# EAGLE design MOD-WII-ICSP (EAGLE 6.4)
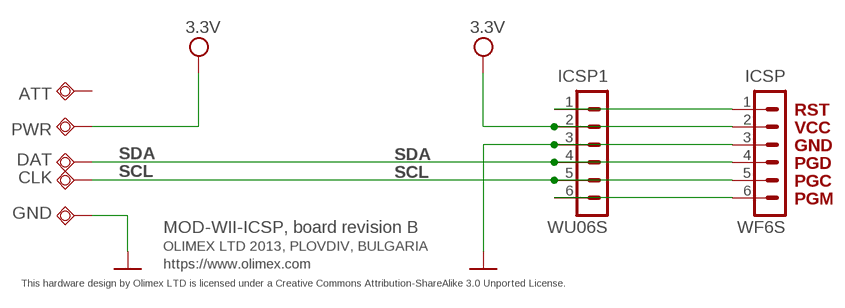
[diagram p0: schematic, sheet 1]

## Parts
ATT  TESTPADTESTPAD1.50X7.5MM  [TESTPAD1.50X7.5MM]
CLK  TESTPADTESTPAD1.50X7.5MM  [TESTPAD1.50X7.5MM]
DAT  TESTPADTESTPAD1.50X7.5MM  [TESTPAD1.50X7.5MM]
GND  TESTPADTESTPAD1.50X7.5MM  [TESTPAD1.50X7.5MM]
ICSP  WF6S  CON6WF6S  [WF6S]
ICSP1  WU06S  CON6WUO6S  [WU06S]
PWR  TESTPADTESTPAD1.50X7.5MM  [TESTPAD1.50X7.5MM]

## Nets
GND [pwr]: GND.1(PP) ICSP1.3 ICSP.3
N$1: ICSP1.1 ICSP.1
N$6: ICSP1.6 ICSP.6
SCL: CLK.1(PP) ICSP1.5 ICSP.5
SDA: DAT.1(PP) ICSP1.4 ICSP.4
VCC: ICSP1.2 ICSP.2 PWR.1(PP) ; supply symbol labelled 3.3V
Unconnected: ATT.1(PP)

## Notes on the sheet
- RST
- VCC
- GND
- PGD
- PGC
- PGM
- MOD-WII-ICSP, board revision B
- OLIMEX LTD 2013, PLOVDIV, BULGARIA
- https://www.olimex.com
- This hardware design by Olimex LTD is licensed under a Creative Commons Attribution-ShareAlike 3.0 Unported License.

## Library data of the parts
ATT CLK DAT GND PWR = gogo:TESTPAD: drill 40mils, diameter 70mils
ICSP ICSP1 = Penko:CON6: CONNECTORS - 6 PINS

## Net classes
1 pwr: width 0.25 mm

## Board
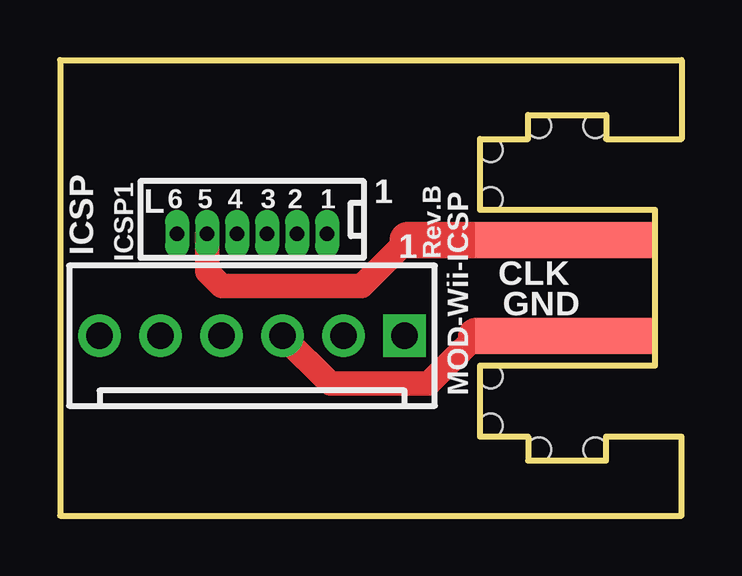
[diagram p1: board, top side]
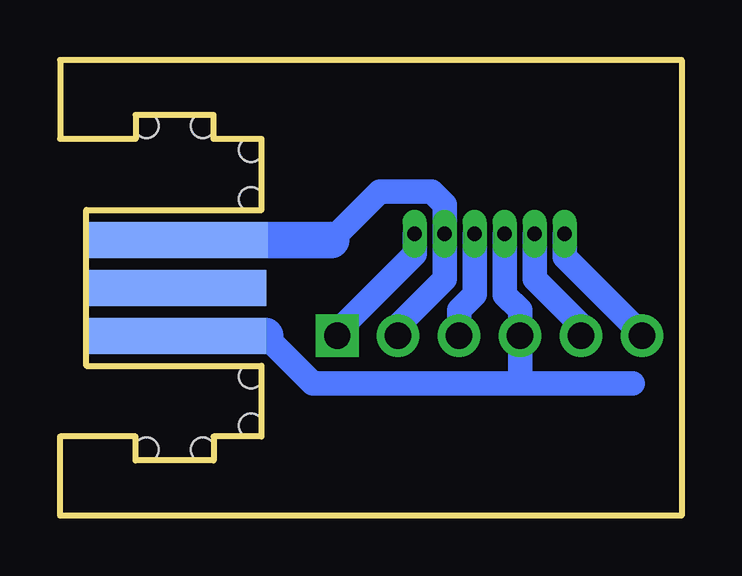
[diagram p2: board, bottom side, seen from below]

Size 25.9 x 19 mm. Coordinates in mm from the lower left corner, seen from the top.
Outline: 17.5,3.3 17.5,6.25 24.8,6.25 24.8,12.75 17.5,12.75 17.5,15.7 19.5,15.7 19.5,16.7 22.75,16.7 22.75,15.7 25.9,15.7 25.9,19 0,19 0,0 25.9,0 25.9,3.3 22.75,3.3 22.75,2.3 19.5,2.3 19.5,3.3 17.5,3.3
Copper layers (1+16): Top 0.035mm / dielectric 1.5mm / Bottom 0.035mm
Design rules "default": minimum track width 0.2mm, minimum drill 0.4mm, track to track 0.25mm, track to pad 0.25mm, pad to pad 0.25mm, via to via 0.25mm, smd to smd 1mil, copper to edge 10mil, drill to drill 8mil, minimum pad ring 8mil, minimum via ring 0.2mm, stop-mask expansion 4mil, vias tented up to drill 25mil, thermal gap 20mil
Holes 1 mm at 19.95,16.25 22.3,16.25 17.95,15.25 17.95,13.2 17.95,5.8 17.95,3.75 19.95,2.75 22.3,2.75

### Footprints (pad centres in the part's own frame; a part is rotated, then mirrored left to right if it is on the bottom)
TESTPAD1.50X7.5MM = smd 7.5 x 1.5: 1 0,0
WF6S = drill 1.1 pad 1.778 square: 1 -6.35,0 | drill 1.1 pad 1.778: 2 -3.81,0; 3 -1.27,0; 4 1.27,0; 5 3.81,0; 6 6.35,0
WU06S = drill 0.6 pad 0.991 long: 1 -3.125,0; 2 -1.875,0; 3 -0.625,0; 4 0.625,0; 5 1.875,0; 6 3.125,0

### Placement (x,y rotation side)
ATT  21.05,9.5 180 bottom
CLK  21.05,11.5 180 top
DAT  21.05,7.5 0 bottom
GND  21.05,7.5 0 top
ICSP  8,7.5 180 top
ICSP1  8,11.75 180 top
PWR  21,11.5 180 bottom

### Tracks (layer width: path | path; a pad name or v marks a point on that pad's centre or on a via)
GND
  Top 1.016: 17.35,7.5 15.37,5.52 11.25,5.52 ICSP.3
  Top 1.524: 17.35,7.5 GND.1
  Bottom 1.016: ICSP1.3 8.62,9.21 9.27,8.56 ICSP.3
N$1
  Bottom 1.016: ICSP1.1 11.12,10.9 14.35,7.68 ICSP.1
N$6
  Bottom 1.016: ICSP1.6 4.88,10.77 1.65,7.55 ICSP.6
SCL
  Top 1.016: 14.49,11.5 12.57,9.58 6.73,9.58 6.12,10.19 ICSP1.5
  Top 1.524: 14.49,11.5 CLK.1
  Bottom 1.016: ICSP1.5 6.12,9.86 4.19,7.93 ICSP.5
SDA
  Bottom 1.016: ICSP1.4 7.38,9.21 6.73,8.56 ICSP.4 6.73,7.29 6.73,5.52 | 17.35,7.5 15.37,5.52 6.73,5.52 | 6.73,5.52 6.1,5.52 | 2.03,5.52 6.73,5.52
  Bottom 1.524: 17.35,7.5 DAT.1
VCC
  Bottom 1.016: ICSP.2 11.81,7.93 9.88,9.87 ICSP1.2 9.88,12.98 10.41,13.52 12.57,13.52 14.59,11.5
  Bottom 1.524: 14.59,11.5 PWR.1

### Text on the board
tNames: 1 | 1 | Rev.B | MOD-Wii-ICSP
bStop: WWW.OLIMEX.COM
